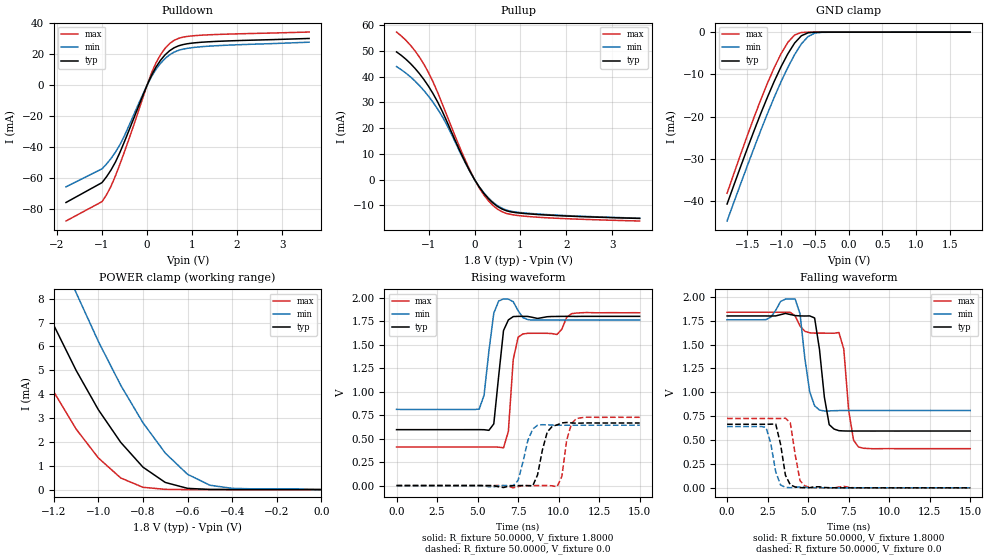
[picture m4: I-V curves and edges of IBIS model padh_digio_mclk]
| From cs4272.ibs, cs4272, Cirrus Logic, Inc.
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|   Model mclk
[Model]  padh_digio_mclk
Model_type I/O
Polarity   Non-Inverting
Enable   Active-High
Vinl =   0.6250V
Vinh =   0.9750V
C_comp   5.0000pF   5.0000pF   5.0000pF
[Temperature Range]   25.0000   85.0000   -40.0000
[Voltage Range]   1.8000V   1.6200V   1.9800V
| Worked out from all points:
|   slope of the pulldown table from 0 to 0.27 V, typ, clamps not added: 18.2 ohm
|   slope of the pullup table from 0 to 0.27 V, typ, clamps not added: 39.9 ohm
|   GND clamp passes 1 mA (typ) near -0.71 V on its own axis
|   POWER clamp passes 1 mA (typ) near -0.81 V on its own axis
|   rising waveform, R_fixture 50.0000, V_fixture 1.8000: 20-80 % time 438ps typ, 378ps min, 521ps max; typ from 0.595 V to 1.8 V
|   rising waveform, R_fixture 50.0000, V_fixture 0.0: 20-80 % time 519ps typ, 572ps min, 426ps max; typ from 0 V to 0.666 V
|   falling waveform, R_fixture 50.0000, V_fixture 1.8000: 20-80 % time 520ps typ, 448ps min, 586ps max; typ from 1.8 V to 0.595 V
|   falling waveform, R_fixture 50.0000, V_fixture 0.0: 20-80 % time 407ps typ, 477ps min, 432ps max; typ from 0.666 V to 0 V
[Pulldown]
|Voltage   I(typ)   I(min)   I(max)
-1.8V     -75.65mA   -65.54mA   -87.6mA
-1V       -62.82mA   -53.93mA   -75.1mA
-900mV    -59.07mA   -50.81mA   -70.72mA
-800mV    -54.68mA   -47.26mA   -65.17mA
-600mV    -43.2mA    -38.24mA   -50.73mA
-100mV    -7.132mA   -6.254mA   -8.793mA
100mV     6.434mA    5.61mA     7.989mA
300mV     16.15mA    14.17mA    19.75mA
500mV     22.27mA    19.65mA    26.88mA
700mV     25.47mA    22.55mA    30.3mA
1.1V      27.52mA    24.61mA    32.13mA
3.6V      30.22mA    27.81mA    34.37mA
[Pullup]
|Voltage   I(typ)   I(min)   I(max)
-1.7V     49.68mA    43.96mA    57.42mA
-1.4V     45.22mA    40.01mA    52.35mA
-1.1V     38.85mA    34.58mA    44.78mA
-900mV    33.31mA    29.96mA    37.86mA
-700mV    26.44mA    24.4mA     29.28mA
-300mV    10.43mA    10.01mA    11.62mA
0V        0A         0A         0A
200mV     -5.305mA   -5.08mA    -5.942mA
500mV     -10.49mA   -10.16mA   -11.53mA
700mV     -12.2mA    -11.92mA   -13.23mA
1.1V      -13.26mA   -13.03mA   -14.3mA
3.6V      -15.16mA   -15.06mA   -16.16mA
[GND_clamp]
|Voltage   I(typ)   I(min)   I(max)
-1.8V     -40.65mA   -44.66mA   -38.1mA
-1.5V     -27.51mA   -31.59mA   -24.45mA
-1.3V     -19.19mA   -23.19mA   -15.94mA
-1.1V     -11.57mA   -15.34mA   -8.334mA
-1V       -8.147mA   -11.68mA   -5.087mA
-900mV    -5.122mA   -8.339mA   -2.404mA
-800mV    -2.577mA   -5.312mA   -665.9uA
-700mV    -855.3uA   -2.776mA   -80.74uA
-600mV    -147.4uA   -1.026mA   -5.602uA
-500mV    -13.65uA   -233.7uA   -1.287uA
-400mV    -1.484uA   -50.98uA   -906.2nA
1.8V      662.4nA    25.4uA     803nA
[POWER_clamp]
|Voltage   I(typ)   I(min)   I(max)
-1.8V     21.57mA    26.57mA    17.86mA
-1.4V     11.23mA    15.41mA    7.973mA
-1.3V     8.972mA    12.88mA    5.919mA
-1.2V     6.884mA    10.49mA    4.094mA
-1.1V     4.998mA    8.253mA    2.537mA
-1V       3.345mA    6.206mA    1.326mA
-900mV    1.982mA    4.376mA    488uA
-800mV    939.9uA    2.8mA      96.54uA
-700mV    299.6uA    1.531mA    10.29uA
-600mV    52.45uA    640.9uA    1.354uA
-400mV    988.9nA    51.76uA    804.8nA
0V        0A         0A         0A
[Ramp]
| variable   typ   min   max
dV/dt_r  0.3993/0.4674n   0.2953/0.6586n   0.5474/0.3912n
dV/dt_f  0.7231/0.4497n   0.5315/0.5845n   0.9226/0.3085n
R_load = 50.0000
[Rising Waveform]
R_fixture= 50.0000
V_fixture= 1.8000
V_fixture_min= 1.9800
V_fixture_max= 1.6200
|time   V(typ)   V(min)   V(max)
0s        594.8mV    810.2mV    410.3mV
5.1ns     594.8mV    813.9mV    410.3mV
5.4ns     594.1mV    961.3mV    410.4mV
5.7ns     587.6mV    1.432V     410.4mV
6ns       656.4mV    1.834V     410.4mV
6.6ns     1.649V     1.986V     401.7mV
6.9ns     1.762V     1.983V     577.1mV
7.2ns     1.798V     1.956V     1.341V
7.5ns     1.8V       1.861V     1.578V
15ns      1.8V       1.76V      1.838V
[Rising Waveform]
R_fixture= 50.0000
V_fixture= 0.0
|time   V(typ)   V(min)   V(max)
0s        0V         115.4uV    0V
7.2ns     -801.9uV   494.5uV    -24.28mV
7.5ns     -122.2uV   54.95mV    -10.89mV
8.4ns     -3.541mV   600.8mV    -114.6uV
9.3ns     570.3mV    645.3mV    159.1uV
9.9ns     645.4mV    642.4mV    -12.56mV
10.2ns    666.2mV    642mV      97.68mV
10.5ns    671.5mV    641.8mV    486.1mV
11.1ns    663mV      641.9mV    713.5mV
15ns      665.5mV    641.9mV    726.2mV
[Falling Waveform]
R_fixture= 50.0000
V_fixture= 1.8000
V_fixture_min= 1.9800
V_fixture_max= 1.6200
|time   V(typ)   V(min)   V(max)
0s        1.8V       1.76V      1.839V
4.2ns     1.804V     1.976V     1.8V
5.1ns     1.8V       1.004V     1.623V
5.4ns     1.779V     859mV      1.62V
6.3ns     661.7mV    805.4mV    1.619V
6.6ns     615.4mV    807.6mV    1.619V
7.2ns     595.7mV    809.6mV    1.453V
7.5ns     594.8mV    809.8mV    814mV
8.1ns     594.9mV    809.8mV    428.3mV
15ns      594.8mV    809.8mV    410.3mV
[Falling Waveform]
R_fixture= 50.0000
V_fixture= 0.0
|time   V(typ)   V(min)   V(max)
0s        665.5mV    641.7mV    726.2mV
2.4ns     665.3mV    632.9mV    726.2mV
2.7ns     666.6mV    462.1mV    726.2mV
3ns       668.3mV    168.4mV    726.2mV
3.3ns     456mV      29.42mV    725.7mV
3.6ns     132mV      5.152mV    729.2mV
3.9ns     31.12mV    1.085mV    681.5mV
4.5ns     2.34mV     9.57mV     74.94mV
4.8ns     504.2uV    6.554mV    19.32mV
15ns      -3.695uV   0V         919.4nV
